| TEXAS INSTRUMENTS INCORPORATED
| Standard Linear and Logic Group
| IBIS Model of SN74VMEH22501
| 8-BIT UNIVERSAL BUS TRANSCEIVERS AND TWO 1-BIT BUS TRANSCEIVERS
| WITH SPLIT LVTTL PORT FEEDBACK PATHS, AND 3-STATE OUTPUTS
| This file contains package information for the following:
|  TSSOP 48-pin (DGG) package as [Component] VMEH22501_DGG
|  TVSOP 48-pin (DGV) package as [Component] VMEH22501_DGV
|  VFBGA 48-pin (GQL) package as [Component] VMEH22501_GQL
| This device can be powered at the following Vccs:
|  3.3 volt Vcc
| This file provides unique models under the [Model Selector] for each Vcc.
| For operation at a specific Vcc, select the appropriate model after each
| [Model Selector] keyword.
[IBIS Ver]   3.2
[Comment char]  |_char
[File Name]   sn74vmeh22501.ibs
[File Rev]   1.1 | x_die
[Date]   April 4, 2002
[Source]   Data created from TI-SPICE simulations at TI-SLL.
[Notes]   The following is an IBIS list for the VMEH22501.
   Please contact sllibis@ti.com with questions and
   comments concerning SLL IBIS models.
   - Since this device can tollerate 5 V signal with
   3.3V VCC, we have some non-monotonic warnings in the pull-up
   curves.
   - As there is no power clamp diode in the Input model,
   we removed the Pwr Clamp table data from the Input models
   - Due to series resistor at the LVTTL port, there is non-
   monotonocity in the pull-up curves
   - Due to over voltage tollerant issue, there is non-monotonocity
   in the ETL side pull-up curves
   - Due to BUS-HOLD Circuit, there is non-monotonic
   warnings in TTL side GND Clamp curve.
[Disclaimer] Property of Texas Instruments Incorporated.  Unauthorized
   reproduction and/or distribution is strictly prohibited.
   This product is protected under copyright law.
   Created  2002, (C) Copyright  2002, Texas Instruments
   Incorporated, All Rights Reserved
   UNLESS THERE IS A SIGNED, WRITTEN AGREEMENT TO THE
   CONTRARY, TEXAS INSTRUMENTS (TI) IS PROVIDING THE IBIS
   MODELS  AND WITHOUT ANY WARRANTY, EXPRESSED OR
   IMPLIED.  TI assumes no liability for:
   1) the accuracy of the IBIS models provided to your
   company;
   2) the proper functioning of these IBIS Models in your
   design or for any resulting applications; or
   3) infringement of patents, copyrights or intellectual
   property rights resulting from your use of these IBIS
   models.
   TI provides IBIS Models as a service to our customers.
   You and your company shall not distribute, sell or give
   these models to anyone else without prior written
   permission from TI.
   TI reserves the right to make changes to our products or
   to discontinue any semiconductor product or service
   without notice, and advises our customers to obtain the
   latest version of relevant information to verify, before
   placing orders, that the information being relied on is
   current.
   Please be aware that your receipt and use of the IBIS
   information provided shall serve as acceptance of these
   terms and conditions.  If you do not accept these terms,
   you should return or destroy the IBIS models and any
   other accompanying information immediately.
| Component VMEH22501_DGG 48-pin TSSOP
[Component]   VMEH22501_DGG
[Manufacturer]   Texas Instruments, Inc.
[Package]
|   typ   min   max
R_pkg   6.200e-02   5.000e-02   7.800e-02
L_pkg   3.527e-09   3.128e-09   4.255e-09
C_pkg   5.300e-13   4.170e-13   6.850e-13
[Pin]   signal_name   model_name   R_pin   L_pin   C_pin
1   1NOEBY   VME_IN_NOEBY   5.000e-02   4.250e-09   6.710e-13
2   1A   VMEH22501_IN_A   5.700e-02   3.956e-09   6.740e-13
3   1Y   VMEH22501_OUT_Y   7.100e-02   3.922e-09   6.190e-13
4   GND   GND   7.800e-02   3.841e-09   6.180e-13
5   2A   VMEH22501_IN_A   5.600e-02   3.535e-09   5.550e-13
6   2Y   VMEH22501_OUT_Y   5.800e-02   3.464e-09   5.030e-13
7   VCC   POWER   6.000e-02   3.362e-09   4.980e-13
8   2NOEBY   VME_IN_NOEBY   6.100e-02   3.293e-09   4.620e-13
9   3A1   VMEH22501_IO_3A   6.300e-02   3.240e-09   4.550e-13
10   GND   GND   6.300e-02   3.175e-09   4.420e-13
11   LE   VMEH22501_IN_LE   6.400e-02   3.153e-09   4.290e-13
12   3A2   VMEH22501_IO_3A   6.500e-02   3.128e-09   4.180e-13
13   3A3   VMEH22501_IO_3A   6.500e-02   3.128e-09   4.180e-13
14   NOE   VME_IN_NOE   6.400e-02   3.154e-09   4.290e-13
15   GND   GND   6.300e-02   3.174e-09   4.420e-13
16   3A4   VMEH22501_IO_3A   6.300e-02   3.241e-09   4.550e-13
17   CLKBA   VME_IN_CLKBA   6.100e-02   3.293e-09   4.620e-13
18   VCC   POWER   6.000e-02   3.362e-09   4.970e-13
19   3A5   VMEH22501_IO_3A   5.800e-02   3.464e-09   5.030e-13
20   3A6   VMEH22501_IO_3A   5.600e-02   3.537e-09   5.600e-13
21   GND   GND   7.700e-02   3.839e-09   6.260e-13
22   3A7   VMEH22501_IO_3A   7.100e-02   3.917e-09   6.270e-13
23   3A8   VMEH22501_IO_3A   5.800e-02   3.955e-09   6.850e-13
24   DIR   VME_IN_DIR   5.200e-02   4.255e-09   6.790e-13
25   VCC   POWER   5.100e-02   4.254e-09   6.760e-13
26   3B8   VMEH22501_IO_3B   5.800e-02   3.957e-09   6.790e-13
27   3B7   VMEH22501_IO_3B   7.100e-02   3.920e-09   6.210e-13
28   GND   GND   7.800e-02   3.843e-09   6.220e-13
29   3B6   VMEH22501_IO_3B   5.600e-02   3.539e-09   5.600e-13
30   3B5   VMEH22501_IO_3B   5.800e-02   3.466e-09   5.030e-13
31   VCC   POWER   6.000e-02   3.363e-09   4.970e-13
32   CLKAB   VME_IN_CLKAB   6.100e-02   3.294e-09   4.620e-13
33   3B4   VMEH22501_IO_3B   6.300e-02   3.241e-09   4.540e-13
34   GND   GND   6.300e-02   3.175e-09   4.410e-13
35   VCC   POWER   6.400e-02   3.153e-09   4.290e-13
36   3B3   VMEH22501_IO_3B   6.500e-02   3.129e-09   4.170e-13
37   3B2   VMEH22501_IO_3B   6.500e-02   3.129e-09   4.170e-13
38   VCC   POWER   6.400e-02   3.152e-09   4.290e-13
39   GND   GND   6.400e-02   3.176e-09   4.410e-13
40   3B1   VMEH22501_IO_3B   6.300e-02   3.241e-09   4.540e-13
41   2OEAB   VME_IN_OEAB   6.100e-02   3.293e-09   4.620e-13
42   VCC   POWER   6.000e-02   3.363e-09   4.970e-13
43   2B   VMEH22501_IO_B   5.800e-02   3.464e-09   5.030e-13
44   BIASVCC   VME_IN_BIAS   5.600e-02   3.534e-09   5.610e-13
45   GND   GND   7.800e-02   3.841e-09   6.260e-13
46   1B   VMEH22501_IO_B   7.100e-02   3.920e-09   6.220e-13
47   VCC   POWER   5.700e-02   3.955e-09   6.770e-13
48   1OEAB   VME_IN_OEAB   5.100e-02   4.252e-09   6.720e-13
| Component VMEH22501_GQL 48-pin VFBGA
[Component]   VMEH22501_GQL
[Manufacturer]   Texas Instruments, Inc.
[Package]
|   typ   min   max
R_pkg   7.90E-02   4.50E-02   9.40E-02
L_pkg   2.26E-09   1.40E-09   2.72E-09
C_pkg   3.06E-13   1.17E-13   4.04E-13
[Pin]   signal_name   model_name   R_pin   L_pin   C_pin
A1   1NOEBY  VME_IN_NOEBY   5.10E-02   1.53E-09   2.10E-13
B2   1A   VMEH22501_IN_A  7.30E-02   2.57E-09   3.12E-13
B1   1Y   VMEH22501_OUT_Y 7.10E-02   1.84E-09   2.32E-13
B3   GND   GND   9.40E-02   2.72E-09   3.83E-13
C2   2A   VMEH22501_IN_A  8.90E-02   2.53E-09   3.50E-13
C1   2Y   VMEH22501_OUT_Y 7.10E-02   1.83E-09   2.31E-13
C3   VCC   POWER   9.40E-02   2.72E-09   3.92E-13
D2   2NOEBY  VME_IN_NOEBY   9.00E-02   2.55E-09   3.52E-13
D1   3A1   VMEH22501_IO_3A 7.20E-02   1.85E-09   2.44E-13
D3   GND   GND   9.40E-02   2.72E-09   4.03E-13
E2   LE   VMEH22501_IN_LE 8.90E-02   2.54E-09   3.51E-13
E1   3A2   VMEH22501_IO_3A 7.20E-02   1.85E-09   2.27E-13
F1   3A3   VMEH22501_IO_3A 7.20E-02   1.85E-09   2.27E-13
F2   NOE   VME_IN_NOE   8.90E-02   2.54E-09   3.51E-13
G3   GND   GND   9.40E-02   2.72E-09   4.04E-13
G1   3A4   VMEH22501_IO_3A 7.20E-02   1.85E-09   2.44E-13
G2   CLKBA   VME_IN_CLKBA   9.00E-02   2.55E-09   3.52E-13
H3   VCC   POWER   9.40E-02   2.72E-09   3.92E-13
H1   3A5   VMEH22501_IO_3A 7.00E-02   1.83E-09   2.31E-13
H2   3A6   VMEH22501_IO_3A 8.80E-02   2.52E-09   3.50E-13
J3   GND   GND   9.30E-02   2.71E-09   3.82E-13
J1   3A7   VMEH22501_IO_3A 7.10E-02   1.85E-09   2.33E-13
J2   3A8   VMEH22501_IO_3A 5.60E-02   2.61E-09   3.90E-13
K1   DIR   VME_IN_DIR   4.50E-02   1.40E-09   1.17E-13
K6   VCC   POWER   4.50E-02   1.51E-09   1.93E-13
J5   3B8   VMEH22501_IO_3B 5.50E-02   2.49E-09   3.13E-13
J6   3B7   VMEH22501_IO_3B 7.00E-02   1.82E-09   2.30E-13
J4   GND   GND   9.30E-02   2.70E-09   3.82E-13
H5   3B6   VMEH22501_IO_3B 8.90E-02   2.53E-09   3.50E-13
H6   3B5   VMEH22501_IO_3B 7.10E-02   1.83E-09   2.30E-13
H4   VCC   POWER   9.40E-02   2.72E-09   3.91E-13
G5   CLKAB   VME_IN_CLKAB   9.00E-02   2.55E-09   3.52E-13
G6   3B4   VMEH22501_IO_3B 7.20E-02   1.85E-09   2.44E-13
G4   GND   GND   9.40E-02   2.72E-09   4.04E-13
F5   VCC   POWER   8.80E-02   2.51E-09   3.49E-13
F6   3B3   VMEH22501_IO_3B 7.20E-02   1.85E-09   2.27E-13
E6   3B2   VMEH22501_IO_3B 7.10E-02   1.85E-09   2.27E-13
E5   VCC   POWER   8.90E-02   2.53E-09   3.50E-13
D4   GND   GND   9.40E-02   2.72E-09   4.03E-13
D6   3B1   VMEH22501_IO_3B 7.20E-02   1.85E-09   2.43E-13
D5   2OEAB   VME_IN_OEAB   8.90E-02   2.55E-09   3.52E-13
C4   VCC   POWER   9.40E-02   2.72E-09   3.91E-13
C6   2B   VMEH22501_IO_B  7.10E-02   1.83E-09   2.30E-13
C5   BIASVCC VME_IN_BIAS   8.90E-02   2.54E-09   3.50E-13
B4   GND   GND   9.30E-02   2.71E-09   3.82E-13
B6   1B   VMEH22501_IO_B  7.10E-02   1.83E-09   2.27E-13
B5   VCC   POWER   7.30E-02   2.69E-09   3.80E-13
A6   1OEAB   VME_IN_OEAB   5.10E-02   1.42E-09   1.33E-13
| Component VMEH22501_DGV 48-pin TVSOP
[Component]   VMEH22501_DGV
[Manufacturer]   Texas Instruments, Inc.
[Package]
|   typ   min   max
R_pkg   7.000e-02   4.900e-02   8.500e-02
L_pkg   3.013e-09   2.743e-09   3.408e-09
C_pkg   3.710e-13   2.940e-13   5.110e-13
[Pin]   signal_name   model_name   R_pin   L_pin   C_pin
1   1NOEBY   VME_IN_NOEBY   4.900e-02   3.393e-09   4.970e-13
2   1A   VMEH22501_IN_A   6.000e-02   3.250e-09   5.020e-13
3   1Y   VMEH22501_OUT_Y   7.700e-02   3.310e-09   4.510e-13
4   GND   GND   8.500e-02   3.299e-09   4.040e-13
5   2A   VMEH22501_IN_A   8.300e-02   3.136e-09   3.600e-13
6   2Y   VMEH22501_OUT_Y   7.700e-02   3.019e-09   3.630e-13
7   VCC   POWER   6.500e-02   2.882e-09   3.490e-13
8   2NOEBY   VME_IN_NOEBY   6.600e-02   2.829e-09   3.140e-13
9   3A1   VMEH22501_IO_3A   6.700e-02   2.796e-09   3.140e-13
10   GND   GND   6.900e-02   2.754e-09   3.080e-13
11   LE   VMEH22501_IN_LE   7.000e-02   2.753e-09   3.010e-13
12   3A2   VMEH22501_IO_3A   7.100e-02   2.745e-09   2.940e-13
13   3A3   VMEH22501_IO_3A   7.000e-02   2.744e-09   2.940e-13
14   NOE   VME_IN_NOE   7.000e-02   2.754e-09   3.010e-13
15   GND   GND   6.900e-02   2.754e-09   3.080e-13
16   3A4   VMEH22501_IO_3A   6.700e-02   2.796e-09   3.140e-13
17   CLKBA   VME_IN_CLKBA   6.600e-02   2.829e-09   3.140e-13
18   VCC   POWER   6.500e-02   2.883e-09   3.500e-13
19   3A5   VMEH22501_IO_3A   7.500e-02   3.014e-09   3.630e-13
20   3A6   VMEH22501_IO_3A   8.000e-02   3.128e-09   3.580e-13
21   GND   GND   8.400e-02   3.295e-09   4.030e-13
22   3A7   VMEH22501_IO_3A   7.800e-02   3.311e-09   4.520e-13
23   3A8   VMEH22501_IO_3A   6.200e-02   3.259e-09   5.010e-13
24   DIR   VME_IN_DIR   5.200e-02   3.404e-09   4.960e-13
25   VCC   POWER   5.300e-02   3.397e-09   5.050e-13
26   3B8   VMEH22501_IO_3B   6.200e-02   3.249e-09   5.110e-13
27   3B7   VMEH22501_IO_3B   7.700e-02   3.308e-09   4.530e-13
28   GND   GND   8.200e-02   3.289e-09   4.030e-13
29   3B6   VMEH22501_IO_3B   7.800e-02   3.121e-09   3.590e-13
30   3B5   VMEH22501_IO_3B   7.400e-02   3.010e-09   3.630e-13
31   VCC   POWER   6.500e-02   2.883e-09   3.490e-13
32   CLKAB   VME_IN_CLKAB   6.700e-02   2.829e-09   3.140e-13
33   3B4   VMEH22501_IO_3B   6.700e-02   2.795e-09   3.140e-13
34   GND   GND   6.900e-02   2.753e-09   3.070e-13
35   VCC   POWER   7.000e-02   2.753e-09   3.010e-13
36   3B3   VMEH22501_IO_3B   7.000e-02   2.743e-09   2.940e-13
37   3B2   VMEH22501_IO_3B   7.000e-02   2.743e-09   2.940e-13
38   VCC   POWER   7.000e-02   2.753e-09   3.010e-13
39   GND   GND   6.900e-02   2.754e-09   3.070e-13
40   3B1   VMEH22501_IO_3B   6.800e-02   2.797e-09   3.140e-13
41   2OEAB   VME_IN_OEAB   6.700e-02   2.830e-09   3.140e-13
42   VCC   POWER   6.400e-02   2.880e-09   3.490e-13
43   2B   VMEH22501_IO_B   7.200e-02   3.004e-09   3.620e-13
44   BIASVCC   VME_IN_BIAS   7.800e-02   3.121e-09   3.590e-13
45   GND   GND   8.400e-02   3.296e-09   4.030e-13
46   1B   VMEH22501_IO_B   7.700e-02   3.308e-09   4.510e-13
47   VCC   POWER   6.200e-02   3.258e-09   4.990e-13
48   1OEAB   VME_IN_OEAB   5.300e-02   3.408e-09   4.940e-13
| Models and submodels in the file (13): VME_IN_OEAB (Input), VME_IN_DIR (Input), VME_IN_CLKAB (Input), VME_IN_CLKBA (Input), VME_IN_BIAS (Input), VMEH22501_IN_A (Input), VMEH22501_IN_LE (Input), VME_IN_NOEBY (Input), VME_IN_NOE (Input), VMEH22501_OUT_Y (3-state), VMEH22501_IO_3A (I/O), VMEH22501_IO_3B (I/O), VMEH22501_IO_B (I/O)
